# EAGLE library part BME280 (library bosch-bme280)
DIGITAL HUMIDITY, PRESSURE AND TEMPERATURE SENSOR * Digital interface I²C (up to 3.4 MHz) and SPI (3 and 4 wire, up to 10 MHz)* Supply voltage VDD main supply voltage range: 1.71 V to 3.6 V*VDDIO interface voltage range: 1.2 V to 3.6 V Operating range -40…+85 °C, 0…100 % rel. humidity, 300…1100 hPa The library has been designed by Richard Magdycz
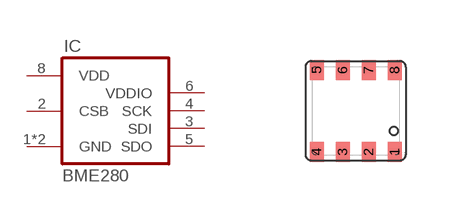
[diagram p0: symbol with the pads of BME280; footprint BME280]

Designator prefix IC

## BME280  [BME280]
1  GND  pwr
2  CSB  in
3  SDI
4  SCK
5  SDO  in
6  VDDIO  pwr
7  GND  pwr
8  VDD  pwr

## Footprint BME280 (pad centres in mm)
2.5 mm x 2.5 mm x 0.93 mm metal lid LGA
smd 0.35 x 0.5: 1 0.975,-1.025; 2 0.325,-1.025; 3 -0.325,-1.025; 4 -0.975,-1.025; 5 -0.975,1.025; 6 -0.325,1.025; 7 0.325,1.025; 8 0.975,1.025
